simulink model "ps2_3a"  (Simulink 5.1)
settings: Solver=ode45  StartTime=0.0  StopTime=10.0  RelTol=1e-3
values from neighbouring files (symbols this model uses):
  s = tf('s')    [ps7_3_2.m]    (also in ps4_2.m; ps7_1_2.m; ps4_3.m; ps2_3.m)
undefined symbols (not defined in the file or in its folder): b
libraries: cstblocks x2

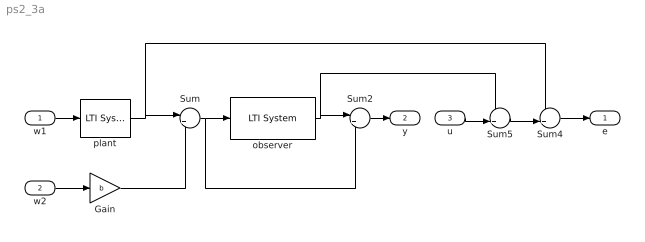
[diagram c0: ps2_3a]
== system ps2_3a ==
  w1 : Inport
  w2 : Inport  Port=2
  u : Inport  Port=3
  Gain : Gain  Gain=b
  Sum : Sum  Inputs=|++
  Sum2 : Sum  Inputs=|+-
  Sum4 : Sum  Inputs=-+|
  Sum5 : Sum  Inputs=++|
  observer : cstblocks/LTI System  sys=(s+1)/(s^2+s+1)  IC=[]
  plant : cstblocks/LTI System  sys=1/s^2  IC=[]
  e : Outport
  y : Outport  Port=2
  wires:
  w1/1 -> plant/1
  w2/1 -> Gain/1
  plant/1 -> Sum/1, Sum4/1
  Gain/1 -> Sum/2
  Sum/1 -> Sum2/2, observer/1
  Sum2/1 -> y/1
  Sum4/1 -> e/1
  u/1 -> Sum5/2
  Sum5/1 -> Sum4/2
  observer/1 -> Sum2/1, Sum5/1
